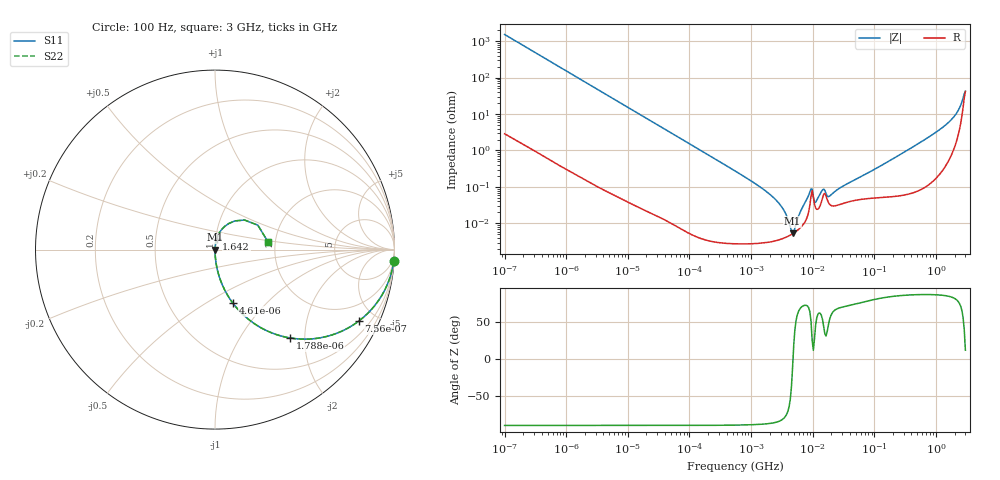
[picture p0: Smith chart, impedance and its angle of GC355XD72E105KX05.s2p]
!Murata Part Number: GC355XD72E105KX05
!These Parameters are Measured in Series Mode Connection
!Data Generated on Jun 10, 2025
!  o--ll--o
!Port1  Port2
!  o------o
!Operation Temp=25[degC], DC Bias Voltage=0[V]
!Freq. Start=100[Hz] Stop=3[GHz] 401[Steps]
# Hz S RI R 50
!Freq.(Hz) S11(Real) S11(Imag) S21(Real) S21(Imag) S12(Real) S12(Imag) S22(Real) S22(Imag)
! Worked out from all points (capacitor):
!   401 points, 100 Hz to 3 GHz, reference 50 ohm
!   read as one part in series: C = 1.05 uF near 109 Hz
!   lowest |Z| = 5.32 mohm at 4.712 MHz (marker M1)
!   series resonance near 4.784 MHz, so ESL is about 1.1 nH
!   S11 on the Smith chart (normalised r, x): 100 Hz: 1, -30; 756 Hz: 1.01, -4.01; 1.788 kHz: 1.00, -1.70; 4.61 kHz: 1.00, -0.66; 1.642 GHz: 1.01, +0.12; 3 GHz: 1.83, +0.17
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100  0.9955 -0.0658  0.00448 0.0658  0.00448 0.0658  0.9955 -0.0658
364  0.9451 -0.2268  0.0549 0.2268  0.0549 0.2268  0.9451 -0.2268
756  0.8004 -0.3987  0.1996 0.3987  0.1996 0.3987  0.8004 -0.3987
1788  0.419 -0.4924  0.581 0.4924  0.581 0.4924  0.419 -0.4924
4610  0.0986 -0.297  0.9014 0.297  0.9014 0.297  0.0986 -0.297
31977  0.00242 -0.0476  0.9976 0.0476  0.9976 0.0476  0.00242 -0.0476
547723  3.53e-05 -0.00276  1 0.00276  1 0.00276  3.53e-05 -0.00276
2266852  3.25e-05 -0.000527  1 0.000527  1 0.000527  3.25e-05 -0.000527
3198641  3.81e-05 -0.000269  1 0.000269  1 0.000269  3.81e-05 -0.000269
4141163  4.61e-05 -9.52e-05  1 9.52e-05  1 9.52e-05  4.61e-05 -9.52e-05
4711951  5.22e-05 -1e-05  0.9999 1e-05  0.9999 1e-05  5.22e-05 -1e-05
5597215  6.41e-05 0.000108  0.9999 -0.000108  0.9999 -0.000108  6.41e-05 0.000108
8986547  0.00032 0.000653  0.9997 -0.000653  0.9997 -0.000653  0.00032 0.000653
9794414  0.00079 0.000365  0.9992 -0.000365  0.9992 -0.000365  0.00079 0.000365
1.11444e7  0.000264 0.000273  0.9997 -0.000273  0.9997 -0.000273  0.000264 0.000273
1.442825e7  0.0005 0.000669  0.9995 -0.000669  0.9995 -0.000669  0.0005 0.000669
1.867972e7  0.000339 0.000444  0.9997 -0.000444  0.9997 -0.000444  0.000339 0.000444
1.751444e8  0.00056 0.00516  0.9994 -0.00516  0.9994 -0.00516  0.00056 0.00516
7.900314e8  0.00179 0.0242  0.9982 -0.0242  0.9982 -0.0242  0.00179 0.0242
1.642185e9  0.00929 0.0603  0.9907 -0.0603  0.9907 -0.0603  0.00929 0.0603
2.419119e9  0.0559 0.1306  0.9441 -0.1306  0.9441 -0.1306  0.0559 0.1306
3e9  0.2951 0.0435  0.7049 -0.0435  0.7049 -0.0435  0.2951 0.0435
